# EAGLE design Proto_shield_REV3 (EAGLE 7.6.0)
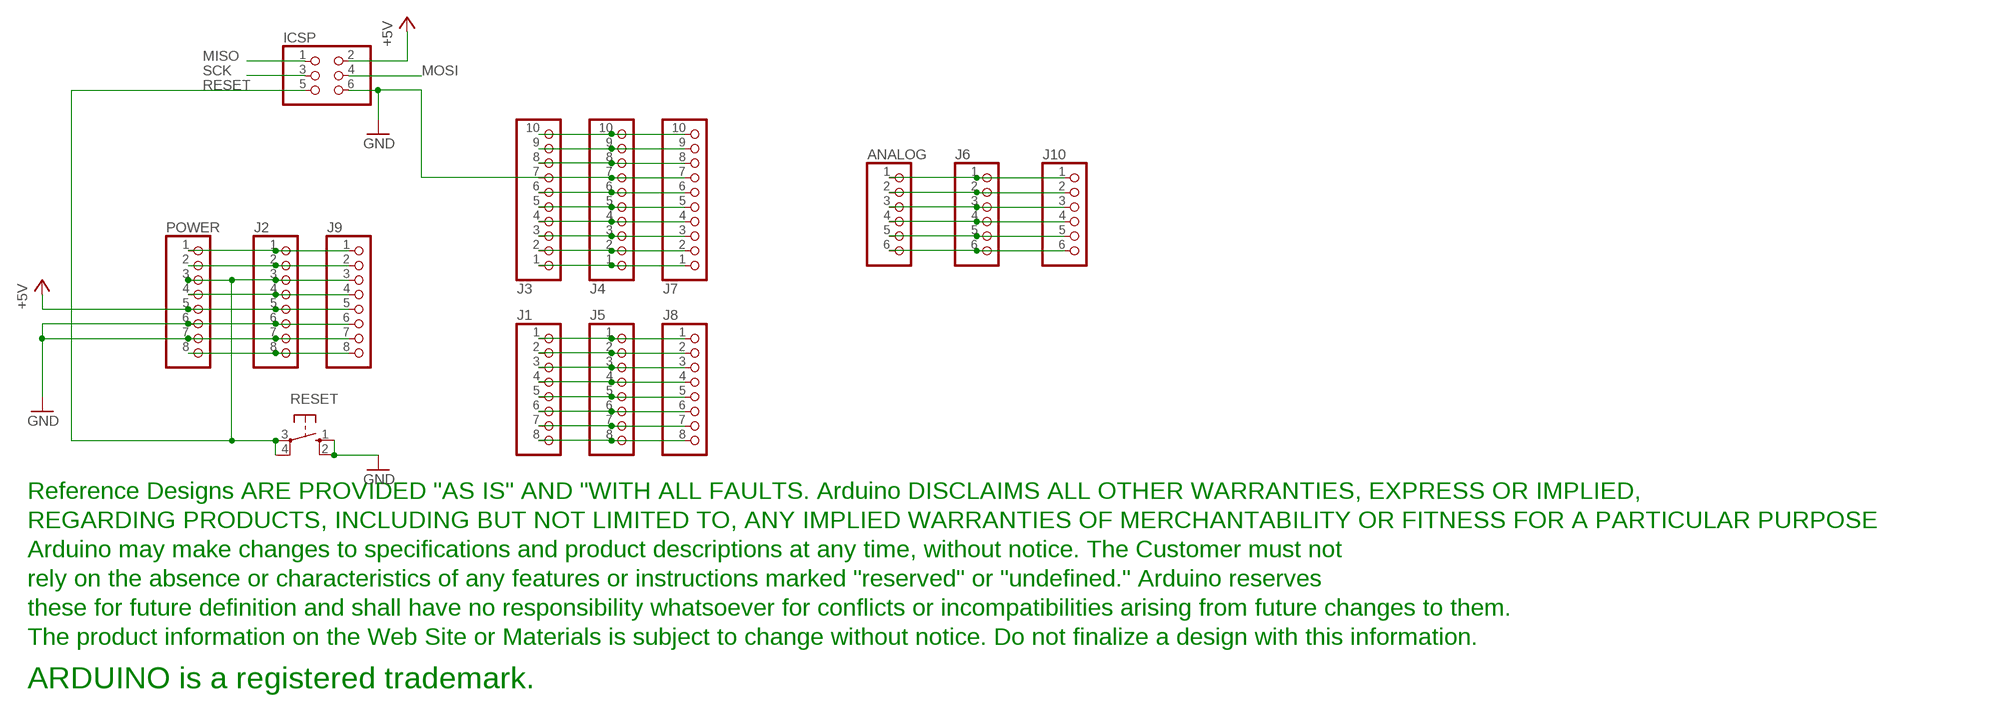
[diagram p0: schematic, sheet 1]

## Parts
ANALOG  PINHD-1X6  [1X06]
ICSP  PINHD-2X3  [2X03]
J1  PINHD-1X8TH  [1X08-TH]
J2  PINHD-1X8TH  [1X08-TH]
J3  PINHD-1X10TH  [1X10-TH]
J4  PINHD-1X10TH  [1X10-TH]
J5  PINHD-1X8TH  [1X08-TH]
J6  PINHD-1X6  [1X06]
J7  PINHD-1X10TH  [1X10-TH]
J8  PINHD-1X8TH  [1X08-TH]
J9  PINHD-1X8TH  [1X08-TH]
J10  PINHD-1X6  [1X06]
POWER  PINHD-1X8TH  [1X08-TH]
RESET  10-XX  [B3F-10XX]
U$1  DISCLAIMER  [DISCLAIMER]

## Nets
+5V: ICSP.2 J2.5 J9.5 POWER.5
+9V: J2.8 J9.8 POWER.8
GND: ICSP.6 J2.6 J2.7 J3.7 J4.7 J7.7 J9.6 J9.7 POWER.6 POWER.7 RESET.1(S) RESET.2(S1)
MISO: ICSP.1
MOSI: ICSP.4
N$1: J3.6 J4.6 J7.6
N$2: J3.1 J4.1 J7.1
N$3: J3.4 J4.4 J7.4
N$4: J3.5 J4.5 J7.5
N$6: J3.2 J4.2 J7.2
N$7: J3.3 J4.3 J7.3
N$8: J1.1 J5.1 J8.1
N$9: J1.2 J5.2 J8.2
N$10: J1.3 J5.3 J8.3
N$11: J1.4 J5.4 J8.4
N$12: J1.5 J5.5 J8.5
N$13: J1.6 J5.6 J8.6
N$14: J1.7 J5.7 J8.7
N$15: J1.8 J5.8 J8.8
N$18: ANALOG.1 J6.1 J10.1
N$19: ANALOG.2 J6.2 J10.2
N$20: ANALOG.3 J6.3 J10.3
N$21: ANALOG.4 J6.4 J10.4
N$22: ANALOG.5 J6.5 J10.5
N$23: ANALOG.6 J6.6 J10.6
N$31: J2.2 J9.2 POWER.2
N$32: J2.1 J9.1 POWER.1
N$141: J3.9 J4.9 J7.9
N$142: J3.10 J4.10 J7.10
N$222: J3.8 J4.8 J7.8
N$223: J2.4 J9.4 POWER.4
RESET: ICSP.5 J2.3 J9.3 POWER.3 RESET.3(P) RESET.4(P1)
SCK: ICSP.3

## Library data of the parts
ANALOG J6 J10 = pinhead:PINHD-1X6: PIN HEADER
ICSP = SmartPrj:PINHD-2X3: PIN HEADER
J1 J2 J5 J8 J9 POWER = SmartPrj:PINHD-1X8: PIN HEADER
J3 J4 J7 = SmartPrj:PINHD-1X10: PIN HEADER
RESET = switch-omron:10-XX: OMRON SWITCH
U$1 = SmartPrj:DISCLAIMER

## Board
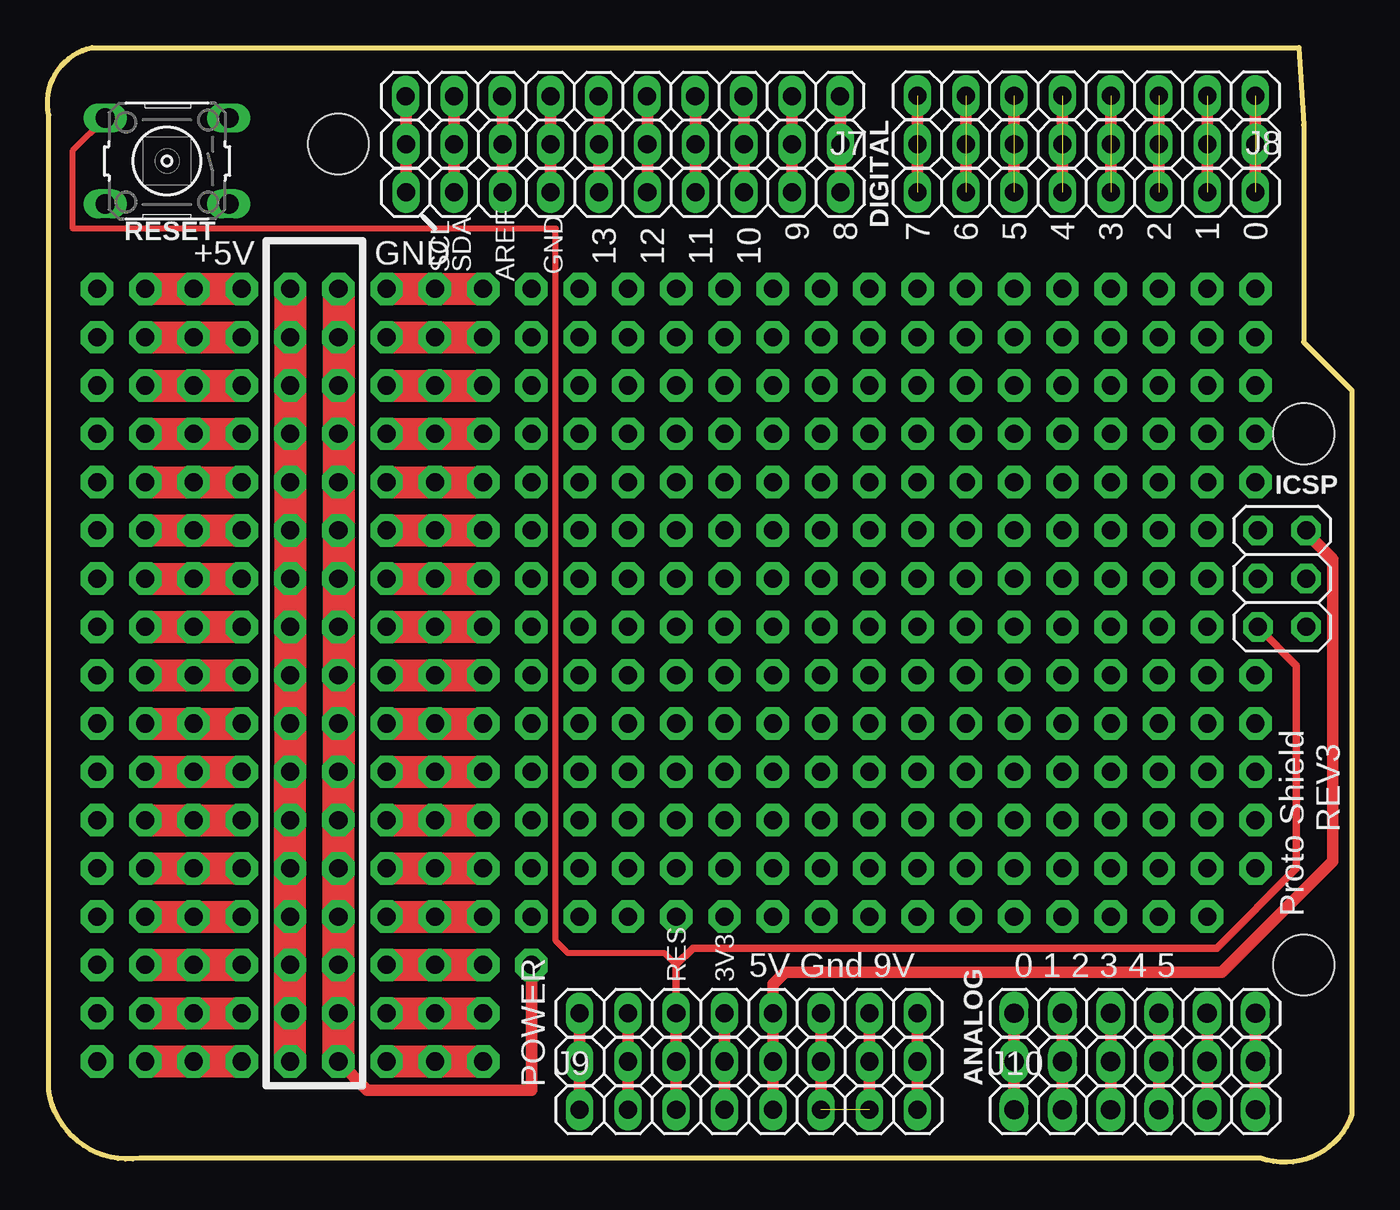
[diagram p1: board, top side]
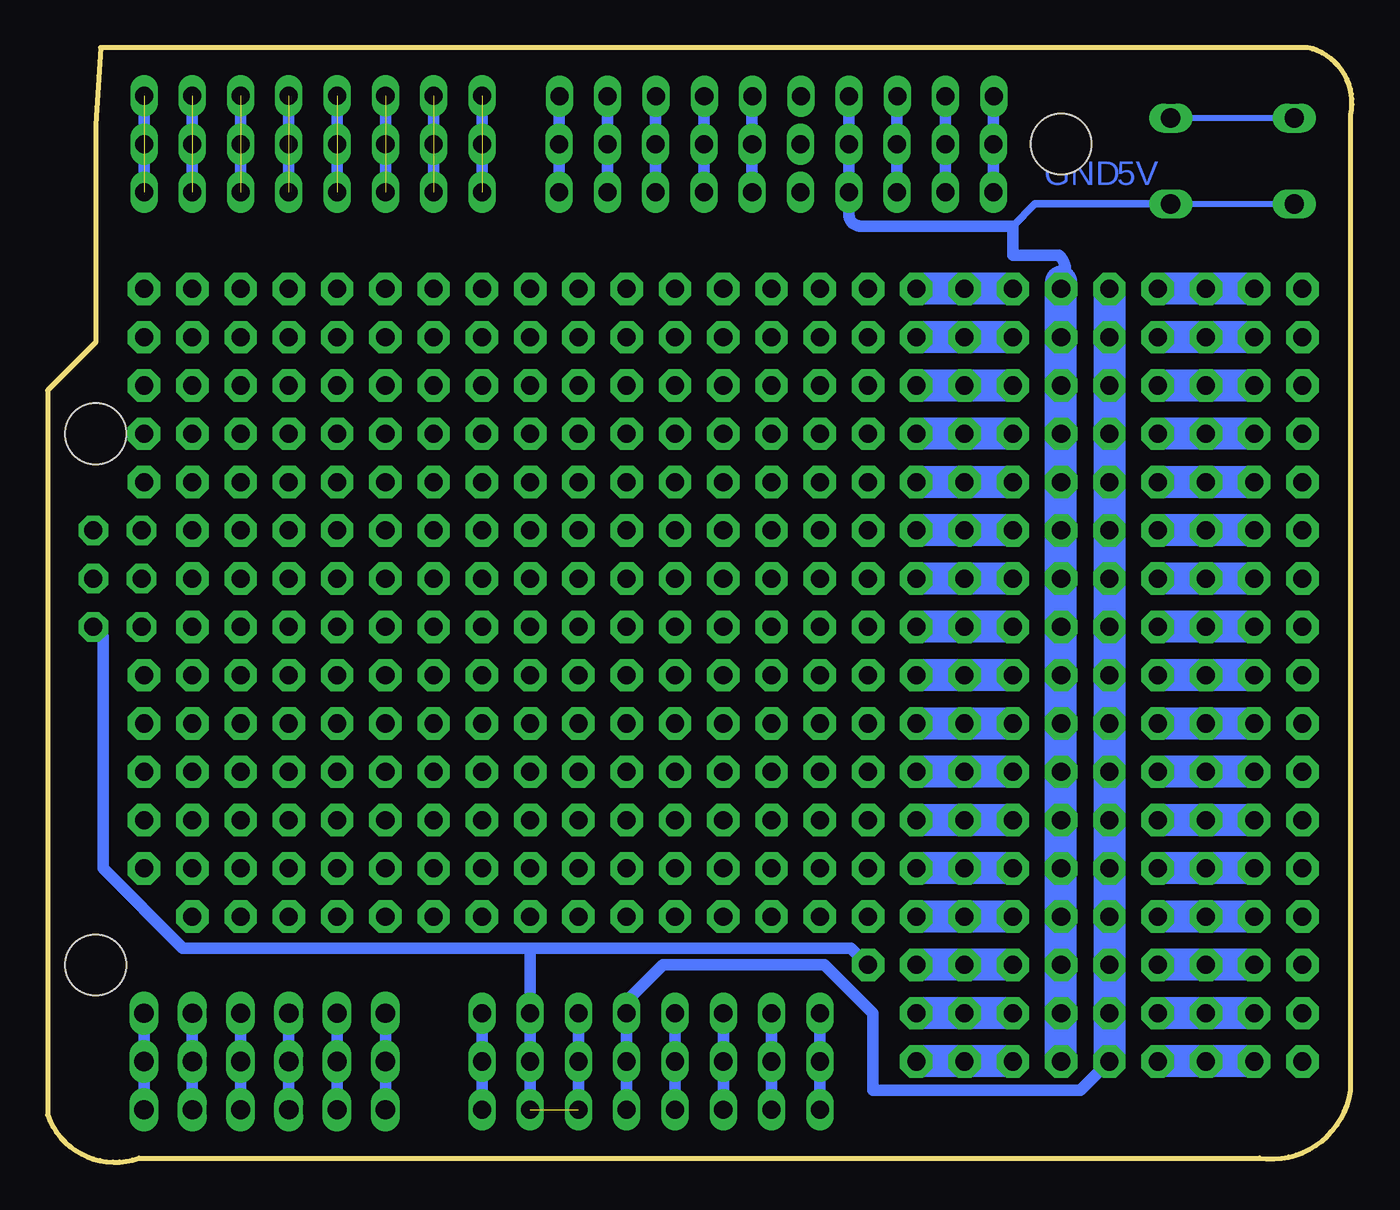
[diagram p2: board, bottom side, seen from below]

Size 68.65 x 58.64 mm. Coordinates in mm from the lower left corner, seen from the top.
Outline: 65.85,58.64 66.11,54.58 66.11,43.15 68.65,40.61 68.65,2.49 arc-90 63.84,0.22 4.88,0.22 arc-90 0.07,3.76 0.07,55.1 arc-90 2.34,58.64 65.85,58.64
Copper layers (1*16): Top 0.035mm / dielectric 1.5mm / Bottom 0.035mm
Design rules "default": minimum track width 10mil, minimum drill 24mil, track to track 8mil, track to pad 8mil, pad to pad 8mil, via to via 8mil, smd to smd 8mil, copper to edge 40mil, drill to drill 8mil, minimum pad ring 10mil, minimum via ring 8mil, stop-mask expansion 2mil, vias tented up to drill 0mil, thermal gap 10mil
Holes 3.2 mm at 15.31,53.56 66.11,10.38 66.11,38.32

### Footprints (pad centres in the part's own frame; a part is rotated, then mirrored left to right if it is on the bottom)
1X06 = drill 1.016 long: 1 -6.35,0; 2 -3.81,0; 3 -1.27,0; 4 1.27,0; 5 3.81,0; 6 6.35,0
2X03 = drill 0.95 pad 1.55 octagon: 1 -2.54,-1.27; 2 -2.54,1.27; 3 0,-1.27; 4 0,1.27; 5 2.54,-1.27; 6 2.54,1.27
1X08-TH = drill 0.95 pad 1.422 long: 1 -8.89,0; 2 -6.35,0; 3 -3.81,0; 4 -1.27,0; 5 1.27,0; 6 3.81,0; 7 6.35,0; 8 8.89,0
1X10-TH = drill 0.95 pad 1.422 long: 1 -11.43,0; 2 -8.89,0; 3 -6.35,0; 4 -3.81,0; 5 -1.27,0; 6 1.27,0; 7 3.81,0; 8 6.35,0; 9 8.89,0; 10 11.43,0
B3F-10XX = drill 1.016 long: 1 -3.251,2.261; 2 3.251,2.261; 3 -3.251,-2.261; 4 3.251,-2.261

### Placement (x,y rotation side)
ANALOG  57.22,5.3 0 top
ICSP  64.96,30.7 270 top
J1  54.68,53.56 180 top
J2  36.9,5.3 0 top
J3  30.29,53.56 180 top
J4  30.29,51.02 180 top
J5  54.68,51.02 180 top
J6  57.22,7.84 0 top
J7  30.28,56.08 180 top
J8  54.68,56.1 180 top
J9  36.9,2.76 0 top
J10  57.22,2.76 0 top
POWER  36.9,7.84 0 top
RESET  6.29,52.67 180 top
U$1  not placed on the board

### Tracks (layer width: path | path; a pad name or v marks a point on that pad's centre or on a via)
+5V  (via drill 0.95 pad 1.7)
  Top 0.61: ICSP.2 66.23,33.11 67.63,31.72 67.63,15.84 61.79,10 38.8,10 38.17,9.36 POWER.5 | 38.17,7.71 J2.5 | 38.17,5.17 J9.5
  Top 1.676: v12.77,5.3 v12.77,7.84 v12.77,10.38 v12.77,12.92 v12.77,15.46 v12.77,18 v12.77,20.54 v12.77,23.08 v12.77,25.62 v12.77,28.16 v12.77,30.7 v12.77,33.24 v12.77,35.78 v12.77,38.32 v12.77,40.86 v12.77,43.4 v12.77,45.94
  Bottom 0.61: v12.77,5.3 14.29,3.78 25.21,3.78 25.21,7.84 27.75,10.38 36.26,10.38 38.17,8.47 POWER.5 J2.5 J9.5
  Bottom 1.676: v12.77,45.94 v12.77,5.3
+9V
  Top 0.61: POWER.8 J2.8 J9.8
  Bottom 0.61: POWER.8 J2.8 J9.8
GND  (via drill 0.95 pad 1.7)  (1 unrouted)
  Top 0.61: v15.31,5.3 16.83,3.78 25.47,3.78 v25.47,10.38 | POWER.7 J2.7 J9.7 | J7.7 26.48,56.1 J3.7 | POWER.6 J2.6 J9.6
  Top 1.676: v15.31,5.3 v15.31,7.84 v15.31,10.38 v15.31,12.92 v15.31,15.46 v15.31,18 v15.31,20.54 v15.31,23.08 v15.31,25.62 v15.31,28.16 v15.31,30.7 v15.31,33.24 v15.31,35.78 v15.31,38.32 v15.31,40.86 v15.31,43.4 v15.31,45.94
  Bottom 0.305: RESET.1 RESET.2
  Bottom 0.406: RESET.1 16.68,50.41 17.85,49.24
  Bottom 0.61: v25.47,10.38 26.36,11.27 43.25,11.27 | 43.25,11.27 61.54,11.27 65.73,15.46 65.73,27.65 ICSP.6 | 43.25,11.27 POWER.7 J2.7 J9.7 | 15.31,46.32 arc-90 15.43,47.72 17.85,47.72 17.85,49.24 25.85,49.24 arc90 26.48,49.88 J4.7 J3.7 26.48,56.1 | POWER.6 J2.6 J9.6
  Bottom 1.676: v15.31,5.3 15.31,46.32
N$1
  Top 0.61: J7.6 29.02,56.1 J3.6 J4.6
N$2
  Top 0.61: 41.72,53.69 J3.1 | J3.1 J4.1 | J7.1 41.72,56.1 J3.1
  Bottom 0.61: J4.1 J3.1 41.72,56.1
N$3
  Top 0.61: 34.1,53.69 J3.4 | J3.4 J4.4 | J7.4 34.1,56.1 J3.4
  Bottom 0.61: J4.4 J3.4 34.1,56.1
N$4
  Top 0.61: J4.5 J3.5 31.56,56.1 J7.5
  Bottom 0.61: J4.5 J3.5 31.56,56.1
N$5
  Top 0.61: 26.48,53.69 26.48,51.15
N$6
  Top 0.61: 39.18,53.69 J3.2 | J3.2 J4.2 | J7.2 39.18,56.1 J3.2
  Bottom 0.61: J3.2 J4.2 J3.2 | J3.2 39.18,56.1
N$7
  Top 0.61: 36.64,53.69 J3.3 | J3.3 J4.3 | J7.3 36.64,56.1 J3.3
  Bottom 0.61: J4.3 J3.3 36.64,56.1
N$8  (1 unrouted)
  Top 0.61: J5.1 J1.1 J8.1
  Bottom 0.61: J5.1 J1.1
N$9  (1 unrouted)
  Top 0.61: J5.2 J1.2 J8.2
  Bottom 0.61: J5.2 J1.2 J8.2 | 63.57,53.56 63.57,56.1
N$10  (1 unrouted)
  Top 0.61: J5.3 J1.3 J8.3
  Bottom 0.61: J5.3 J1.3 J8.3
N$11  (1 unrouted)
  Top 0.61: J5.4 J1.4 J8.4
  Bottom 0.61: J5.4 J1.4 J8.4
N$12  (1 unrouted)
  Top 0.61: J5.5 J1.5 J8.5
  Bottom 0.61: J5.5 J1.5 J8.5
N$13  (1 unrouted)
  Top 0.61: J5.6 J1.6 J8.6
  Bottom 0.61: J5.6 J1.6 J8.6
N$14  (1 unrouted)
  Top 0.61: J5.7 J1.7 J8.7
  Bottom 0.61: J5.7 J1.7 J8.7
N$15  (1 unrouted)
  Top 0.61: 45.79,53.69 J1.8 | J1.8 J5.8 | 45.79,56.23 J1.8
  Bottom 0.61: J5.8 J1.8 J8.8
N$16  (via drill 0.95 pad 1.7)
  other vias: 50.87,33.24
N$17  (via drill 0.95 pad 1.7)
  other vias: 53.41,25.62
N$18
  Top 0.61: J6.1 ANALOG.1 J10.1
  Bottom 0.61: J6.1 ANALOG.1 J10.1
N$19
  Top 0.61: J6.2 ANALOG.2 J10.2
  Bottom 0.61: J6.2 ANALOG.2 J10.2
N$20
  Top 0.61: J6.3 ANALOG.3 J10.3
  Bottom 0.61: J6.3 ANALOG.3 J10.3
N$21
  Top 0.61: J6.4 ANALOG.4 J10.4
  Bottom 0.61: J6.4 ANALOG.4 J10.4
N$22
  Top 0.61: J6.5 ANALOG.5 J10.5
  Bottom 0.61: J6.5 ANALOG.5 J10.5
N$23
  Top 0.61: J6.6 ANALOG.6 J10.6
  Bottom 0.61: J6.6 ANALOG.6 J10.6
N$26  (via drill 0.95 pad 1.7)
  other vias: 53.41,30.7
N$27  (via drill 0.95 pad 1.7)
  Top 1.676: v17.85,7.84 v22.93,7.84
N$28  (via drill 0.95 pad 1.7)
  other vias: 20.39,7.84
N$31
  Top 0.61: POWER.2 J2.2 J9.2
  Bottom 0.61: POWER.2 J2.2 J9.2
N$32
  Top 0.61: POWER.1 J2.1 J9.1
  Bottom 0.61: POWER.1 J2.1 J9.1
N$33  (via drill 0.95 pad 1.7)
  other vias: 7.69,7.84
N$34  (via drill 0.95 pad 1.7)
  Top 1.676: v5.15,7.84 v10.23,7.84
N$36  (via drill 0.95 pad 1.7)
  other vias: 20.39,10.38
N$37  (via drill 0.95 pad 1.7)
  Top 1.676: v17.85,10.38 v22.93,10.38
N$38  (via drill 0.95 pad 1.7)
  other vias: 55.95,30.7
N$39  (via drill 0.95 pad 1.7)
  other vias: 58.49,33.24
N$40  (via drill 0.95 pad 1.7)
  other vias: 30.55,30.7
N$41  (via drill 0.95 pad 1.7)
  Top 1.676: v5.15,10.38 v10.23,10.38
N$42  (via drill 0.95 pad 1.7)
  other vias: 7.69,10.38
N$43  (via drill 0.95 pad 1.7)
  other vias: 58.49,30.7
N$44  (via drill 0.95 pad 1.7)
  other vias: 33.09,30.7
N$45  (via drill 0.95 pad 1.7)
  other vias: 45.79,12.92
N$46  (via drill 0.95 pad 1.7)
  other vias: 28.01,12.92
N$47  (via drill 0.95 pad 1.7)
  other vias: 25.47,12.92
N$48  (via drill 0.95 pad 1.7)
  Top 1.676: v17.85,12.92 v22.93,12.92
N$49  (via drill 0.95 pad 1.7)
  other vias: 20.39,12.92
N$50  (via drill 0.95 pad 1.7)
  other vias: 55.95,28.16
N$51  (via drill 0.95 pad 1.7)
  other vias: 58.49,28.16
N$52  (via drill 0.95 pad 1.7)
  other vias: 55.95,25.62
N$53  (via drill 0.95 pad 1.7)
  other vias: 53.41,28.16
N$54  (via drill 0.95 pad 1.7)
  other vias: 7.69,12.92
N$55  (via drill 0.95 pad 1.7)
  Top 1.676: v5.15,12.92 v10.23,12.92
N$56  (via drill 0.95 pad 1.7)
  other vias: 2.61,7.84
N$57  (via drill 0.95 pad 1.7)
  other vias: 53.41,15.46
N$58  (via drill 0.95 pad 1.7)
  other vias: 28.01,15.46
N$59  (via drill 0.95 pad 1.7)
  other vias: 25.47,15.46
N$60
  Bottom 1.676: 17.85,7.84 22.93,7.84
N$61  (via drill 0.95 pad 1.7)
  other vias: 20.39,15.46
N$62  (via drill 0.95 pad 1.7)
  Top 1.676: v17.85,15.46 v22.93,15.46
N$63  (via drill 0.95 pad 1.7)
  other vias: 22.93,30.7
N$64  (via drill 0.95 pad 1.7)
  other vias: 22.93,33.24
N$65  (via drill 0.95 pad 1.7)
  Top 1.676: v5.15,15.46 v10.23,15.46
N$66  (via drill 0.95 pad 1.7)
  other vias: 7.69,15.46
N$67  (via drill 0.95 pad 1.7)
  Top 1.676: v5.15,25.62 v10.23,25.62
N$68  (via drill 0.95 pad 1.7)
  other vias: 35.63,28.16
N$69  (via drill 0.95 pad 1.7)
  other vias: 43.25,18
N$70  (via drill 0.95 pad 1.7)
  other vias: 28.01,18
N$71  (via drill 0.95 pad 1.7)
  other vias: 25.47,18
N$72  (via drill 0.95 pad 1.7)
  Top 1.676: v17.85,18 v22.93,18
N$73  (via drill 0.95 pad 1.7)
  other vias: 20.39,18
N$74  (via drill 0.95 pad 1.7)
  other vias: 7.69,25.62
N$75  (via drill 0.95 pad 1.7)
  other vias: 7.69,23.08
N$76  (via drill 0.95 pad 1.7)
  Top 1.676: v22.93,25.62 v20.39,25.62 v17.85,25.62
N$77  (via drill 0.95 pad 1.7)
  Top 1.676: v22.93,23.08 v20.39,23.08 v17.85,23.08
N$78  (via drill 0.95 pad 1.7)
  other vias: 7.69,18
N$79  (via drill 0.95 pad 1.7)
  Top 1.676: v5.15,18 v10.23,18
N$80  (via drill 0.95 pad 1.7)
  other vias: 35.63,30.7
N$81  (via drill 0.95 pad 1.7)
  other vias: 58.49,20.54
N$82  (via drill 0.95 pad 1.7)
  other vias: 28.01,20.54
N$83  (via drill 0.95 pad 1.7)
  other vias: 25.47,20.54
N$84  (via drill 0.95 pad 1.7)
  Top 1.676: v5.15,20.54 v10.23,20.54
N$85  (via drill 0.95 pad 1.7)
  other vias: 20.39,20.54
N$86  (via drill 0.95 pad 1.7)
  Top 1.676: v17.85,20.54 v22.93,20.54
N$87  (via drill 0.95 pad 1.7)
  Top 1.676: v5.15,23.08 v10.23,23.08
N$88  (via drill 0.95 pad 1.7)
  other vias: 22.93,35.78
N$89  (via drill 0.95 pad 1.7)
  other vias: 22.93,38.32
N$90  (via drill 0.95 pad 1.7)
  other vias: 7.69,20.54
N$91  (via drill 0.95 pad 1.7)
  other vias: 22.93,40.86
N$92  (via drill 0.95 pad 1.7)
  other vias: 38.17,28.16
N$93  (via drill 0.95 pad 1.7)
  other vias: 61.03,23.08
N$94  (via drill 0.95 pad 1.7)
  other vias: 28.01,23.08
N$95  (via drill 0.95 pad 1.7)
  other vias: 25.47,23.08
N$96  (via drill 0.95 pad 1.7)
  other vias: 22.93,43.4
N$97  (via drill 0.95 pad 1.7)
  other vias: 38.17,30.7
N$98  (via drill 0.95 pad 1.7)
  other vias: 40.71,28.16
N$99  (via drill 0.95 pad 1.7)
  other vias: 40.71,30.7
N$100  (via drill 0.95 pad 1.7)
  other vias: 43.25,30.7
N$101  (via drill 0.95 pad 1.7)
  other vias: 45.79,30.7
N$102  (via drill 0.95 pad 1.7)
  other vias: 48.33,30.7
N$103  (via drill 0.95 pad 1.7)
  other vias: 50.87,30.7
N$104  (via drill 0.95 pad 1.7)
  other vias: 50.87,28.16
N$105  (via drill 0.95 pad 1.7)
  other vias: 63.57,25.62
N$106  (via drill 0.95 pad 1.7)
  other vias: 28.01,25.62
N$107  (via drill 0.95 pad 1.7)
  other vias: 25.47,25.62
N$108  (via drill 0.95 pad 1.7)
  other vias: 22.93,45.94
N$109  (via drill 0.95 pad 1.7)
  other vias: 48.33,28.16
N$110  (via drill 0.95 pad 1.7)
  other vias: 43.25,28.16
N$111  (via drill 0.95 pad 1.7)
  other vias: 30.55,28.16
N$112
  Bottom 1.676: 17.85,30.7 22.93,30.7
N$113  (via drill 0.95 pad 1.7)
  Top 1.676: v17.85,30.7 22.93,30.7
N$114
  Bottom 1.676: 5.15,45.94 10.23,45.94
N$115
  Bottom 1.676: 17.85,43.4 22.93,43.4
N$116
  Bottom 1.676: 17.85,25.62 22.93,25.62
N$117  (via drill 0.95 pad 1.7)
  other vias: 61.03,28.16
N$118  (via drill 0.95 pad 1.7)
  Top 1.676: v17.85,28.16 v20.39,28.16 v22.93,28.16
N$119  (via drill 0.95 pad 1.7)
  other vias: 28.01,28.16
N$120  (via drill 0.95 pad 1.7)
  other vias: 25.47,28.16
N$121
  Bottom 1.676: 17.85,23.08 22.93,23.08
N$122
  Bottom 1.676: 17.85,20.54 22.93,20.54
N$123  (via drill 0.95 pad 1.7)
  other vias: 25.47,45.94
N$124
  Bottom 1.676: 17.85,18 22.93,18
N$125
  Bottom 1.676: 17.85,15.46 22.93,15.46
N$126
  Bottom 1.676: 17.85,12.92 22.93,12.92
N$127
  Bottom 1.676: 5.15,7.84 10.23,7.84
N$128
  Bottom 1.676: 5.15,12.92 10.23,12.92
N$129
  Bottom 1.676: 5.15,15.46 10.23,15.46
N$130
  Bottom 1.676: 5.15,18 10.23,18
N$131  (via drill 0.95 pad 1.7)
  other vias: 28.01,30.7
N$132  (via drill 0.95 pad 1.7)
  other vias: 25.47,30.7
N$133
  Bottom 1.676: 5.15,20.54 10.23,20.54
N$134
  Bottom 1.676: 5.15,23.08 10.23,23.08
N$135  (via drill 0.95 pad 1.7)
  other vias: 25.47,33.24
N$136
  Bottom 1.676: 5.15,25.62 10.23,25.62 | 5.15,28.16 10.23,28.16 | 5.15,30.7 10.23,30.7 | 5.15,33.24 10.23,33.24 | 5.15,35.78 10.23,35.78
N$137
  Bottom 1.676: 5.15,10.38 10.23,10.38
N$138
  Bottom 1.676: 5.15,5.3 10.23,5.3
N$139
  Bottom 1.676: 17.85,10.38 22.93,10.38
N$140
  Bottom 1.676: 17.85,5.3 22.93,5.3
N$141
  Top 0.61: 21.4,53.69 J3.9 | J3.9 J4.9 | J7.9 21.4,56.1 J3.9
  Bottom 0.61: J4.9 J3.9 21.4,56.1
N$142
  Top 0.61: 18.86,53.69 J3.10 | J3.10 J4.10 | J7.10 18.86,56.1 J3.10
  Bottom 0.61: J4.10 J3.10 18.86,56.1
N$143  (via drill 0.95 pad 1.7)
  other vias: 28.01,33.24
N$144  (via drill 0.95 pad 1.7)
  other vias: 20.39,35.78
N$145
  Bottom 1.676: 17.85,35.78 22.93,35.78
N$146
  Bottom 1.676: 17.85,38.32 22.93,38.32
N$147  (via drill 0.95 pad 1.7)
  other vias: 2.61,45.94
N$148  (via drill 0.95 pad 1.7)
  other vias: 2.61,43.4
N$149  (via drill 0.95 pad 1.7)
  other vias: 2.61,40.86
N$150  (via drill 0.95 pad 1.7)
  other vias: 2.61,38.32
N$151  (via drill 0.95 pad 1.7)
  other vias: 2.61,35.78
N$152  (via drill 0.95 pad 1.7)
  other vias: 2.61,33.24
N$153  (via drill 0.95 pad 1.7)
  other vias: 55.95,35.78
N$154  (via drill 0.95 pad 1.7)
  other vias: 2.61,30.7
N$155  (via drill 0.95 pad 1.7)
  other vias: 28.01,35.78
N$156  (via drill 0.95 pad 1.7)
  other vias: 25.47,35.78
N$157  (via drill 0.95 pad 1.7)
  other vias: 2.61,28.16
N$158  (via drill 0.95 pad 1.7)
  other vias: 2.61,25.62
N$159  (via drill 0.95 pad 1.7)
  other vias: 2.61,23.08
N$160  (via drill 0.95 pad 1.7)
  other vias: 2.61,20.54
N$161  (via drill 0.95 pad 1.7)
  other vias: 2.61,18
N$162  (via drill 0.95 pad 1.7)
  other vias: 2.61,15.46
N$163  (via drill 0.95 pad 1.7)
  other vias: 2.61,12.92
N$164  (via drill 0.95 pad 1.7)
  other vias: 2.61,10.38
N$165  (via drill 0.95 pad 1.7)
  other vias: 50.87,38.32
N$166  (via drill 0.95 pad 1.7)
  other vias: 2.61,5.3
N$167  (via drill 0.95 pad 1.7)
  other vias: 28.01,38.32
N$168  (via drill 0.95 pad 1.7)
  other vias: 25.47,38.32
N$169  (via drill 0.95 pad 1.7)
  other vias: 7.69,30.7
N$170  (via drill 0.95 pad 1.7)
  Top 1.676: v5.15,30.7 v10.23,30.7
N$171  (via drill 0.95 pad 1.7)
  Top 1.676: v5.15,28.16 v10.23,28.16
N$172  (via drill 0.95 pad 1.7)
  other vias: 7.69,33.24
N$173  (via drill 0.95 pad 1.7)
  Top 1.676: v5.15,33.24 v10.23,33.24
N$174  (via drill 0.95 pad 1.7)
  Top 1.676: v5.15,35.78 v10.23,35.78
N$175  (via drill 0.95 pad 1.7)
  other vias: 7.69,35.78
N$176
  Bottom 1.676: 5.15,38.32 10.23,38.32
N$177  (via drill 0.95 pad 1.7)
  other vias: 43.25,40.86
N$178  (via drill 0.95 pad 1.7)
  Top 1.676: v17.85,40.86 22.93,40.86
N$179  (via drill 0.95 pad 1.7)
  other vias: 28.01,40.86
N$180  (via drill 0.95 pad 1.7)
  other vias: 25.47,40.86
N$181  (via drill 0.95 pad 1.7)
  other vias: 7.69,38.32
N$182
  Bottom 1.676: 5.15,40.86 10.23,40.86
N$183  (via drill 0.95 pad 1.7)
  other vias: 7.69,40.86
N$184  (via drill 0.95 pad 1.7)
  Top 1.676: v5.15,40.86 v10.23,40.86
N$185  (via drill 0.95 pad 1.7)
  Top 1.676: v5.15,38.32 v10.23,38.32
N$186  (via drill 0.95 pad 1.7)
  Top 1.676: v5.15,43.4 v10.23,43.4
N$187  (via drill 0.95 pad 1.7)
  other vias: 7.69,43.4
N$188
  Bottom 1.676: 5.15,43.4 10.23,43.4
N$189  (via drill 0.95 pad 1.7)
  other vias: 63.57,43.4
N$190  (via drill 0.95 pad 1.7)
  other vias: 7.69,28.16
N$191  (via drill 0.95 pad 1.7)
  other vias: 28.01,43.4
N$192  (via drill 0.95 pad 1.7)
  other vias: 25.47,43.4
N$193  (via drill 0.95 pad 1.7)
  other vias: 7.69,45.94
N$194  (via drill 0.95 pad 1.7)
  Top 1.676: v5.15,45.94 v10.23,45.94
N$195  (via drill 0.95 pad 1.7)
  Top 1.676: v17.85,45.94 22.93,45.94
N$196  (via drill 0.95 pad 1.7)
  other vias: 20.39,45.94
N$197  (via drill 0.95 pad 1.7)
  other vias: 20.39,43.4
N$198
  Bottom 1.676: 17.85,45.94 22.93,45.94
N$199  (via drill 0.95 pad 1.7)
  Top 1.676: v17.85,43.4 22.93,43.4
N$200
  Bottom 1.676: 17.85,40.86 22.93,40.86
N$201  (via drill 0.95 pad 1.7)
  other vias: 38.17,45.94
N$202  (via drill 0.95 pad 1.7)
  Top 1.676: v17.85,33.24 22.93,33.24
N$203  (via drill 0.95 pad 1.7)
  other vias: 28.01,45.94
N$204
  Bottom 1.676: 17.85,33.24 22.93,33.24
N$205  (via drill 0.95 pad 1.7)
  other vias: 20.39,33.24
N$206  (via drill 0.95 pad 1.7)
  other vias: 20.39,30.7
N$207
  Bottom 1.676: 17.85,28.16 22.93,28.16
N$208  (via drill 0.95 pad 1.7)
  Top 1.676: v17.85,35.78 22.93,35.78
N$209  (via drill 0.95 pad 1.7)
  Top 1.676: v17.85,38.32 22.93,38.32
N$210  (via drill 0.95 pad 1.7)
  other vias: 20.39,38.32
N$211  (via drill 0.95 pad 1.7)
  other vias: 20.39,40.86
N$222
  Top 0.61: 23.94,53.69 J3.8 | J3.8 J4.8 23.94,50.89 | J7.8 23.94,56.1 J3.8
  Bottom 0.61: J4.8 J3.8 23.94,56.1
N$223
  Top 0.61: POWER.4 J2.4 J9.4
  Bottom 0.61: POWER.4 J2.4 J9.4
N$227  (via drill 0.95 pad 1.7)
  other vias: 30.55,40.86
N$228  (via drill 0.95 pad 1.7)
  other vias: 33.09,40.86
N$229  (via drill 0.95 pad 1.7)
  other vias: 30.55,38.32
N$230  (via drill 0.95 pad 1.7)
  other vias: 33.09,38.32
N$231  (via drill 0.95 pad 1.7)
  other vias: 30.55,35.78
N$232  (via drill 0.95 pad 1.7)
  other vias: 33.09,35.78
N$233  (via drill 0.95 pad 1.7)
  other vias: 35.63,38.32
N$234  (via drill 0.95 pad 1.7)
  other vias: 35.63,35.78
N$235  (via drill 0.95 pad 1.7)
  other vias: 33.09,33.24
N$236  (via drill 0.95 pad 1.7)
  other vias: 35.63,33.24
N$237  (via drill 0.95 pad 1.7)
  other vias: 38.17,35.78
N$238  (via drill 0.95 pad 1.7)
  other vias: 38.17,38.32
N$239  (via drill 0.95 pad 1.7)
  other vias: 38.17,33.24
N$240  (via drill 0.95 pad 1.7)
  other vias: 40.71,35.78
N$241  (via drill 0.95 pad 1.7)
  other vias: 40.71,38.32
N$242  (via drill 0.95 pad 1.7)
  other vias: 38.17,40.86
N$243  (via drill 0.95 pad 1.7)
  other vias: 35.63,40.86
N$245  (via drill 0.95 pad 1.7)
  other vias: 33.09,43.4
N$246  (via drill 0.95 pad 1.7)
  other vias: 35.63,43.4
N$247  (via drill 0.95 pad 1.7)
  other vias: 30.55,43.4
N$248  (via drill 0.95 pad 1.7)
  other vias: 30.55,45.94
N$249  (via drill 0.95 pad 1.7)
  other vias: 33.09,45.94
N$251  (via drill 0.95 pad 1.7)
  other vias: 30.55,33.24
N$252  (via drill 0.95 pad 1.7)
  other vias: 45.79,28.16
N$259  (via drill 0.95 pad 1.7)
  other vias: 33.09,25.62
N$261  (via drill 0.95 pad 1.7)
  other vias: 35.63,25.62
N$262  (via drill 0.95 pad 1.7)
  other vias: 38.17,25.62
N$263  (via drill 0.95 pad 1.7)
  other vias: 40.71,25.62
N$267  (via drill 0.95 pad 1.7)
  other vias: 43.25,33.24
N$268  (via drill 0.95 pad 1.7)
  other vias: 40.71,33.24
N$269  (via drill 0.95 pad 1.7)
  other vias: 45.79,33.24
N$271  (via drill 0.95 pad 1.7)
  other vias: 33.09,28.16
N$272  (via drill 0.95 pad 1.7)
  other vias: 30.55,25.62
N$273  (via drill 0.95 pad 1.7)
  other vias: 30.55,23.08
N$274  (via drill 0.95 pad 1.7)
  other vias: 33.09,18
N$275  (via drill 0.95 pad 1.7)
  other vias: 33.09,20.54
N$276  (via drill 0.95 pad 1.7)
  other vias: 38.17,20.54
N$277  (via drill 0.95 pad 1.7)
  other vias: 35.63,20.54
N$278  (via drill 0.95 pad 1.7)
  other vias: 35.63,18
N$279  (via drill 0.95 pad 1.7)
  other vias: 30.55,18
N$280  (via drill 0.95 pad 1.7)
  other vias: 30.55,20.54
N$281  (via drill 0.95 pad 1.7)
  other vias: 38.17,23.08
N$282  (via drill 0.95 pad 1.7)
  other vias: 40.71,23.08
N$283  (via drill 0.95 pad 1.7)
  other vias: 38.17,18
N$284  (via drill 0.95 pad 1.7)
  other vias: 30.55,15.46
N$285  (via drill 0.95 pad 1.7)
  other vias: 33.09,15.46
N$286  (via drill 0.95 pad 1.7)
  other vias: 30.55,12.92
N$289  (via drill 0.95 pad 1.7)
  other vias: 33.09,12.92
N$290  (via drill 0.95 pad 1.7)
  other vias: 35.63,12.92
N$291  (via drill 0.95 pad 1.7)
  other vias: 35.63,15.46
N$292  (via drill 0.95 pad 1.7)
  other vias: 38.17,15.46
N$293  (via drill 0.95 pad 1.7)
  other vias: 40.71,20.54
N$294  (via drill 0.95 pad 1.7)
  other vias: 43.25,20.54
N$295  (via drill 0.95 pad 1.7)
  other vias: 43.25,23.08
N$296  (via drill 0.95 pad 1.7)
  other vias: 45.79,23.08
N$297  (via drill 0.95 pad 1.7)
  other vias: 45.79,25.62
N$298  (via drill 0.95 pad 1.7)
  other vias: 43.25,25.62
N$299  (via drill 0.95 pad 1.7)
  other vias: 48.33,25.62
N$304  (via drill 0.95 pad 1.7)
  other vias: 53.41,33.24
N$305  (via drill 0.95 pad 1.7)
  other vias: 48.33,33.24
N$307  (via drill 0.95 pad 1.7)
  other vias: 45.79,35.78
N$309  (via drill 0.95 pad 1.7)
  other vias: 50.87,35.78
N$310  (via drill 0.95 pad 1.7)
  other vias: 48.33,35.78
N$311  (via drill 0.95 pad 1.7)
  other vias: 43.25,35.78
N$312  (via drill 0.95 pad 1.7)
  other vias: 43.25,38.32
N$313  (via drill 0.95 pad 1.7)
  other vias: 45.79,38.32
N$314  (via drill 0.95 pad 1.7)
  other vias: 33.09,23.08
N$315  (via drill 0.95 pad 1.7)
  other vias: 35.63,23.08
N$316  (via drill 0.95 pad 1.7)
  other vias: 45.79,20.54
N$317  (via drill 0.95 pad 1.7)
  other vias: 48.33,23.08
N$318  (via drill 0.95 pad 1.7)
  other vias: 50.87,23.08
N$319  (via drill 0.95 pad 1.7)
  other vias: 50.87,25.62
N$320  (via drill 0.95 pad 1.7)
  other vias: 55.95,23.08
N$321  (via drill 0.95 pad 1.7)
  other vias: 63.57,23.08
N$322  (via drill 0.95 pad 1.7)
  other vias: 63.57,20.54
N$323  (via drill 0.95 pad 1.7)
  other vias: 61.03,20.54
N$324  (via drill 0.95 pad 1.7)
  other vias: 63.57,18
N$325  (via drill 0.95 pad 1.7)
  other vias: 63.57,15.46
N$326  (via drill 0.95 pad 1.7)
  other vias: 61.03,15.46
N$327  (via drill 0.95 pad 1.7)
  other vias: 58.49,15.46
N$331  (via drill 0.95 pad 1.7)
  other vias: 7.69,5.3
N$332  (via drill 0.95 pad 1.7)
  Top 1.676: v5.15,5.3 v10.23,5.3
N$335  (via drill 0.95 pad 1.7)
  Top 1.676: v17.85,5.3 v22.93,5.3
N$336  (via drill 0.95 pad 1.7)
  other vias: 20.39,5.3
N$353  (via drill 0.95 pad 1.7)
  other vias: 61.03,12.92
N$354  (via drill 0.95 pad 1.7)
  other vias: 58.49,12.92
N$355  (via drill 0.95 pad 1.7)
  other vias: 55.95,12.92
N$356  (via drill 0.95 pad 1.7)
  other vias: 53.41,12.92
N$357  (via drill 0.95 pad 1.7)
  other vias: 50.87,12.92
N$358  (via drill 0.95 pad 1.7)
  other vias: 48.33,12.92
N$359  (via drill 0.95 pad 1.7)
  other vias: 40.71,12.92
N$360  (via drill 0.95 pad 1.7)
  other vias: 38.17,12.92
N$361  (via drill 0.95 pad 1.7)
  other vias: 43.25,12.92
N$362  (via drill 0.95 pad 1.7)
  other vias: 43.25,15.46
N$363  (via drill 0.95 pad 1.7)
  other vias: 40.71,15.46
N$364  (via drill 0.95 pad 1.7)
  other vias: 45.79,15.46
N$365  (via drill 0.95 pad 1.7)
  other vias: 48.33,15.46
N$366  (via drill 0.95 pad 1.7)
  other vias: 55.95,15.46
N$367  (via drill 0.95 pad 1.7)
  other vias: 50.87,15.46
N$368  (via drill 0.95 pad 1.7)
  other vias: 61.03,18
N$369  (via drill 0.95 pad 1.7)
  other vias: 58.49,18
N$370  (via drill 0.95 pad 1.7)
  other vias: 55.95,18
N$371  (via drill 0.95 pad 1.7)
  other vias: 53.41,18
N$372  (via drill 0.95 pad 1.7)
  other vias: 50.87,18
N$373  (via drill 0.95 pad 1.7)
  other vias: 48.33,18
N$374  (via drill 0.95 pad 1.7)
  other vias: 45.79,18
N$375  (via drill 0.95 pad 1.7)
  other vias: 40.71,18
N$376  (via drill 0.95 pad 1.7)
  other vias: 48.33,20.54
N$377  (via drill 0.95 pad 1.7)
  other vias: 50.87,20.54
N$378  (via drill 0.95 pad 1.7)
  other vias: 53.41,20.54
N$379  (via drill 0.95 pad 1.7)
  other vias: 55.95,20.54
N$380  (via drill 0.95 pad 1.7)
  other vias: 58.49,23.08
N$381  (via drill 0.95 pad 1.7)
  other vias: 53.41,23.08
N$383  (via drill 0.95 pad 1.7)
  other vias: 58.49,25.62
N$385  (via drill 0.95 pad 1.7)
  other vias: 61.03,25.62
N$393  (via drill 0.95 pad 1.7)
  other vias: 61.03,30.7
N$395  (via drill 0.95 pad 1.7)
  other vias: 55.95,33.24
N$396  (via drill 0.95 pad 1.7)
  other vias: 61.03,33.24
N$397  (via drill 0.95 pad 1.7)
  other vias: 63.57,35.78
N$398  (via drill 0.95 pad 1.7)
  other vias: 61.03,35.78
N$399  (via drill 0.95 pad 1.7)
  other vias: 58.49,35.78
N$400  (via drill 0.95 pad 1.7)
  other vias: 53.41,35.78
N$401  (via drill 0.95 pad 1.7)
  other vias: 63.57,38.32
N$402  (via drill 0.95 pad 1.7)
  other vias: 58.49,38.32
N$403  (via drill 0.95 pad 1.7)
  other vias: 61.03,38.32
N$404  (via drill 0.95 pad 1.7)
  other vias: 63.57,40.86
N$405  (via drill 0.95 pad 1.7)
  other vias: 61.03,40.86
N$406  (via drill 0.95 pad 1.7)
  other vias: 58.49,40.86
N$407  (via drill 0.95 pad 1.7)
  other vias: 55.95,40.86
N$408  (via drill 0.95 pad 1.7)
  other vias: 55.95,38.32
N$409  (via drill 0.95 pad 1.7)
  other vias: 53.41,40.86
N$410  (via drill 0.95 pad 1.7)
  other vias: 53.41,38.32
N$411  (via drill 0.95 pad 1.7)
  other vias: 48.33,38.32
N$412  (via drill 0.95 pad 1.7)
  other vias: 50.87,40.86
N$413  (via drill 0.95 pad 1.7)
  other vias: 48.33,40.86
N$414  (via drill 0.95 pad 1.7)
  other vias: 45.79,40.86
N$415  (via drill 0.95 pad 1.7)
  other vias: 40.71,40.86
N$416  (via drill 0.95 pad 1.7)
  other vias: 38.17,43.4
N$417  (via drill 0.95 pad 1.7)
  other vias: 43.25,43.4
N$418  (via drill 0.95 pad 1.7)
  other vias: 40.71,43.4
N$419  (via drill 0.95 pad 1.7)
  other vias: 45.79,43.4
N$420  (via drill 0.95 pad 1.7)
  other vias: 48.33,43.4
N$421  (via drill 0.95 pad 1.7)
  other vias: 50.87,43.4
N$422  (via drill 0.95 pad 1.7)
  other vias: 53.41,43.4
N$423  (via drill 0.95 pad 1.7)
  other vias: 55.95,43.4
N$424  (via drill 0.95 pad 1.7)
  other vias: 58.49,43.4
N$425  (via drill 0.95 pad 1.7)
  other vias: 61.03,43.4
N$426  (via drill 0.95 pad 1.7)
  other vias: 63.57,45.94
N$427  (via drill 0.95 pad 1.7)
  other vias: 61.03,45.94
N$428  (via drill 0.95 pad 1.7)
  other vias: 58.49,45.94
N$429  (via drill 0.95 pad 1.7)
  other vias: 55.95,45.94
N$430  (via drill 0.95 pad 1.7)
  other vias: 50.87,45.94
N$431  (via drill 0.95 pad 1.7)
  other vias: 53.41,45.94
N$432  (via drill 0.95 pad 1.7)
  other vias: 48.33,45.94
N$433  (via drill 0.95 pad 1.7)
  other vias: 45.79,45.94
N$434  (via drill 0.95 pad 1.7)
  other vias: 43.25,45.94
N$435  (via drill 0.95 pad 1.7)
  other vias: 40.71,45.94
N$436  (via drill 0.95 pad 1.7)
  other vias: 35.63,45.94
RESET
  Top 0.305: 33.09,10.38 32.45,11.01 27.37,11.01 26.74,11.65 26.74,49.11 1.34,49.11 1.34,53.23 RESET.4
  Top 0.406: ICSP.5 65.73,26.13 65.73,15.46 61.54,11.27 33.98,11.27 33.09,10.38 33.09,7.97 POWER.3
  Top 0.61: 33.09,7.97 33.09,5.43 | 33.09,5.43 J2.3 | 33.09,5.43 J9.3
  Bottom 0.305: RESET.4 RESET.3
  Bottom 0.61: POWER.3 J2.3 J9.3

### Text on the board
Bottom: 5V | GND
tPlace: 9 | 8 | 7 | 6 | 5 | 4 | 3 | 2 | 1 | 0 | +5V | GND | 13 | 12 | 11 | 10 | REV3 | Proto Shield
tNames: DIGITAL | AREF | SCL | SDA | GND | RES | 3V3 | 5V Gnd 9V | 0 1 2 3 4 5
bStop: DIGITAL | SDA | AREF | SCL | GND | 13 | 12 | 11 | 9 | 8 | 7 | 6 | 5 | 4 | 3 | 2 | 1 | 0 | 10 | 1 | 2 | 3 | 4 | 5 | 6 | IOREF | RST | 3.3V | 5V | GND | GND | VIN | ANALOG | 0 | 1 | 2 | 3 | 4 | 5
